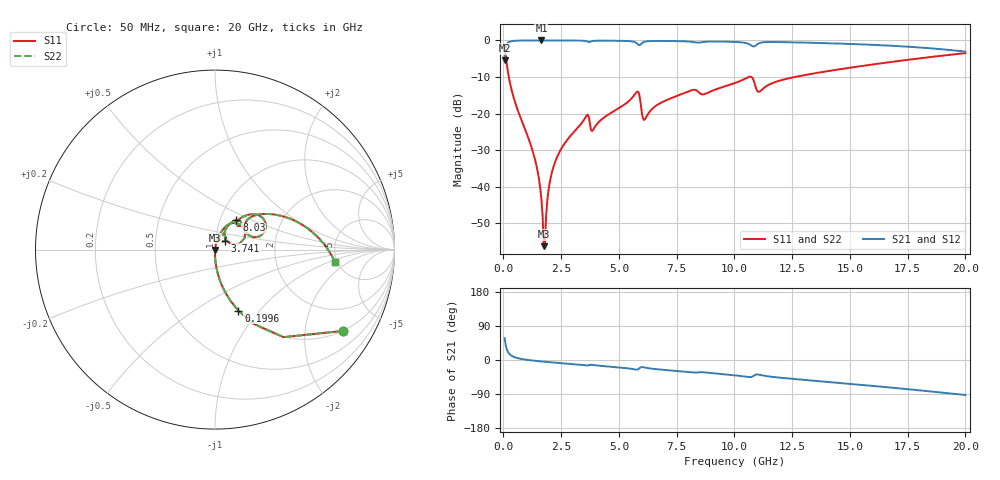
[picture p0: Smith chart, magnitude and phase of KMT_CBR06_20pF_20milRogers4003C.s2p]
! Data measured by Modelithics Inc. support@modelithics.com 813-866-6335
! KEMET CBR0603 20pF, Pad Width= 0.851mm, Pad Length= 0.64mm, Pad Gap= 0.62mm, 20mil Rogers 4003C substrate Data, January 2022
# hz S ma R 50
! 2 Port Network Data from SP1.SP block
! freq  magS11  angS11  magS21  angS21  magS12  angS12  magS22  angS22
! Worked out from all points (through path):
!   401 points, 50 MHz to 20 GHz, reference 50 ohm
!   highest |S21| = -0.01 dB at 1.646 GHz (marker M1); lowest = -5.4 dB at 50 MHz (marker M2)
!   group delay of S21, straight-line fit = 13.2 ps
!   lowest |S11| = -56.2 dB at 1.746 GHz (marker M3), VSWR 1.00, Z = 50.1 - j0.133 ohm
!   |S11| at or under -10 dB: 234 MHz to 10.62 GHz (10.38 GHz wide, 191 % of centre); 10.74 GHz to 12.61 GHz (1.873 GHz wide, 16 % of centre)
!   |S22| runs from -56.2 to -1.5 dB; largest |S21 - S12| = 0
!   S11 on the Smith chart (normalised r, x): 50 MHz: 0.99, -3.15; 199.6 MHz: 0.99, -0.78; 3.741 GHz: 1.11, +0.11; 8.03 GHz: 1.19, +0.41; 20 GHz: 4.78, -1.17
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5e7  0.8449 -32.4  0.5345 57.5  0.5345 57.5  0.8449 -32.4
1.99625e8  0.3642 -69.1  0.9309 20.9  0.9309 20.9  0.3642 -69.1
5.4875e8  0.1294 -83.7  0.9911 6.0  0.9911 6.0  0.1294 -83.7
1.34675e9  0.025 -90.2  0.9989 -2.0  0.9989 -2.0  0.025 -90.2
1.54625e9  0.01232 -89.3  0.999 -3.2  0.999 -3.2  0.01232 -89.3
1.646e9  0.006668 -86.3  0.9991 -3.8  0.9991 -3.8  0.006668 -86.3
1.74575e9  0.001549 -59.0  0.999 -4.4  0.999 -4.4  0.001549 -59.0
1.8455e9  0.00392 71.4  0.999 -4.9  0.999 -4.9  0.00392 71.4
2.045e9  0.01334 79.8  0.9989 -6.0  0.9989 -6.0  0.01334 79.8
2.2445e9  0.02221 80.3  0.9986 -7.0  0.9986 -7.0  0.02221 80.3
3.391625e9  0.07463 73.8  0.9928 -12.9  0.9928 -12.9  0.07463 73.8
3.74075e9  0.0735 40.5  0.9543 -12.9  0.9543 -12.9  0.0735 40.5
5.73575e9  0.1924 49.5  0.9319 -25.3  0.9319 -25.3  0.1924 49.5
6.13475e9  0.08458 47.1  0.9639 -20.1  0.9639 -20.1  0.08458 47.1
6.73325e9  0.1359 62.3  0.9838 -24.9  0.9838 -24.9  0.1359 62.3
8.03e9  0.2023 54.0  0.9651 -32.0  0.9651 -32.0  0.2023 54.0
1.0025e10  0.2624 47.1  0.954 -40.6  0.954 -40.6  0.2624 47.1
1.067338e10  0.3199 31.7  0.877 -45.2  0.877 -45.2  0.3199 31.7
1.107238e10  0.1988 32.1  0.9168 -38.8  0.9168 -38.8  0.1988 32.1
1.336662e10  0.3508 34.5  0.9284 -54.3  0.9284 -54.3  0.3508 34.5
1.670825e10  0.5042 16.0  0.8487 -72.4  0.8487 -72.4  0.5042 16.0
2e10  0.671 -5.7  0.7026 -92.4  0.7026 -92.4  0.671 -5.7
